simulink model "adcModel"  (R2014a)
settings: Solver=ode5  SolverMode=SingleTasking  StartTime=0.0  StopTime=0.3  MaxStep=1/512000  RelTol=1e-3  AbsTol=1e-6
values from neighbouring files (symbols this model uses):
  Wn = Wn_values(i)    [adc_script.m]
undefined symbols (not defined in the file or in its folder): fir1
libraries: dspmlti4 x3, dsparch4 x1, dspmisc x1

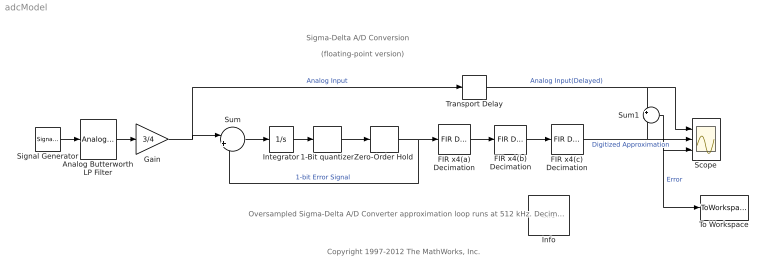
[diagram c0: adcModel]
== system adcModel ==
  note: Oversampled Sigma-Delta A/D Converter approximation loop runs at 512 kHz. Decimation by 64 yields final 8 kHz A/D rate.
  note: Copyright 1997-2012 The MathWorks, Inc.
  note: Sigma-Delta A/D Conversion
  note: (floating-point version)
  1-Bit quantizer : Signum
  Analog Butterworth LP Filter : dsparch4/Analog Filter Design  method=Butterworth  filttype=Lowpass  N=5  Wlo=2*pi*400  Whi=80  Rp=2  Rs=40
  FIR x4(a) Decimation : dspmlti4/FIR Decimation  h=fir1(31,Wn)  D=4  filtStruct=Direct form  framing=Allow multirate processing  inputOffset=0  outputBufInitCond=0  firstCoeffDataTypeStr=Inherit: Same word length as input  firstCoeffLastDataTypeStr=Inherit: Same word length as input  firstCoeffMin=[]  firstCoeffMax=[]  outputMin=[]  outputMax=[]  accumDataTypeStr=Inherit: Same as product output  accumLastDataTypeStr=Inherit: Same as product output  roundingMode=Floor  overflowMode=off  FilterSource=Specify via dialog  FilterObject=Hm_firdecim
  FIR x4(b) Decimation : dspmlti4/FIR Decimation  h=fir1(31,Wn)  D=4  filtStruct=Direct form  framing=Allow multirate processing  inputOffset=0  outputBufInitCond=0  firstCoeffDataTypeStr=Inherit: Same word length as input  firstCoeffLastDataTypeStr=Inherit: Same word length as input  firstCoeffMin=[]  firstCoeffMax=[]  outputMin=[]  outputMax=[]  accumDataTypeStr=Inherit: Same as product output  accumLastDataTypeStr=Inherit: Same as product output  roundingMode=Floor  overflowMode=off  FilterSource=Specify via dialog  FilterObject=Hm_firdecim
  FIR x4(c) Decimation : dspmlti4/FIR Decimation  h=fir1(31,Wn)  D=4  filtStruct=Direct form  framing=Allow multirate processing  inputOffset=0  outputBufInitCond=0  firstCoeffDataTypeStr=Inherit: Same word length as input  firstCoeffLastDataTypeStr=Inherit: Same word length as input  firstCoeffMin=[]  firstCoeffMax=[]  outputMin=[]  outputMax=[]  accumDataTypeStr=Inherit: Same as product output  accumLastDataTypeStr=Inherit: Same as product output  roundingMode=Floor  overflowMode=off  FilterSource=Specify via dialog  FilterObject=Hm_firdecim
  Gain : Gain  Gain=3/4
  Info : dspmisc/Info  SystemSampleTime=-1
  Integrator : Integrator
  Scope : Scope  NumInputPorts=3
  Signal Generator : SignalGenerator  WaveForm=square  Frequency=80
  Sum : Sum  Inputs=|+-
  Sum1 : Sum  Inputs=+-
  To Workspace : ToWorkspace  VariableName=errorArray  SampleTime=-1
  Transport Delay : TransportDelay  DelayTime=336/512000
  Zero-Order Hold : ZeroOrderHold  SampleTime=1/512000
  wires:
  Zero-Order Hold/1 -> FIR x4(a) Decimation/1, Sum/2  "1-bit Error Signal"
  1-Bit quantizer/1 -> Zero-Order Hold/1
  Sum/1 -> Integrator/1
  Integrator/1 -> 1-Bit quantizer/1
  FIR x4(c) Decimation/1 -> Scope/2, Sum1/2  "Digitized Approximation"
  Gain/1 -> Sum/1, Transport Delay/1  "Analog Input"
  Analog Butterworth LP Filter/1 -> Gain/1
  Signal Generator/1 -> Analog Butterworth LP Filter/1
  FIR x4(a) Decimation/1 -> FIR x4(b) Decimation/1
  FIR x4(b) Decimation/1 -> FIR x4(c) Decimation/1
  Sum1/1 -> Scope/3, To Workspace/1  "Error"
  Transport Delay/1 -> Sum1/1, Scope/1  "Analog Input(Delayed)"
